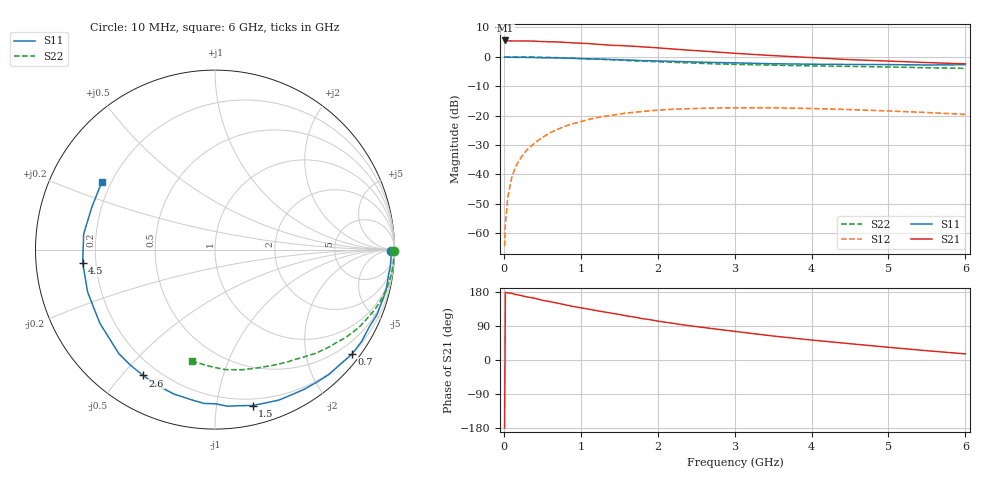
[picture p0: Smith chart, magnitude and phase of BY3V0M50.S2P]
! SIEMENS Small Signal Semiconductors
! BFY420
! Si NPN RF SIEGET Grounded Emitter Transistor in MICRO-X
! VCE = 3 V  IC = 0.5 mA
! Common Emitter S-Parameters:  October  1996
# GHz  S  MA  R  50
!  f  S11  S21  S12  S22
! GHz  MAG  ANG  MAG  ANG  MAG  ANG  MAG  ANG
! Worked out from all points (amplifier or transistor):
!   36 points, 10 MHz to 6 GHz, reference 50 ohm
!   highest |S21| = 5.6 dB at 20 MHz (marker M1)
!   |S21| within 3 dB of that: start of sweep to 2.243 GHz
!   unconditionally stable (mu >= 1): 4.71 GHz to end of sweep
!   at 250 MHz: K = 0.03, MSG = 19.3 dB, |S12| = -33.3 dB
!   at 1.4 GHz: K = 0.17, MSG = 11.9 dB, |S12| = -19.9 dB
!   at 6 GHz: K = 1.43, MAG = 4.7 dB, |S12| = -19.6 dB
!   S11 on the Smith chart (normalised r, x): 10 MHz: 81, -44; 700 MHz: 0.20, -2.96; 1.5 GHz: 0.15, -1.26; 2.6 GHz: 0.14, -0.57; 4.5 GHz: 0.15, -0.05; 6 GHz: 0.16, +0.27
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0.01  0.9811 -0.6  1.891 -179.2  0.0006 87.6  0.9999 -0.3
0.02  0.981 -1.2  1.897 178.8  0.0014 98.1  0.9999 -0.6
0.05  0.9817 -2.8  1.871 177.3  0.004 90.9  0.9999 -1.2
0.1  0.9812 -5.6  1.864 176.1  0.0086 88.0  0.9986 -2.5
0.15  0.9772 -8.1  1.861 172.7  0.0133 84.5  0.9964 -3.7
0.25  0.9793 -13.4  1.864 168.9  0.0217 81.1  0.9948 -6.2
0.4  0.9726 -21.7  1.847 163.0  0.0342 76.7  0.988 -9.9
0.5  0.9611 -26.9  1.813 157.6  0.0424 73.6  0.9821 -12.3
0.7  0.9604 -37.2  1.79 149.9  0.0585 66.8  0.9657 -17.1
0.9  0.9418 -47.6  1.727 141.3  0.0727 60.1  0.9451 -21.6
1.1  0.9231 -57.6  1.681 134.3  0.0858 54.2  0.9234 -25.9
1.5  0.8937 -76.4  1.558 120.2  0.1061 42.8  0.8786 -33.7
1.8  0.8592 -89.7  1.476 109.1  0.1172 35.2  0.8436 -39.0
2.2  0.8368 -105.8  1.356 96.7  0.1281 25.9  0.8072 -45.6
2.6  0.8074 -119.7  1.249 85.7  0.1331 18.1  0.7709 -51.5
3  0.7893 -132.7  1.147 75.6  0.1353 11.4  0.7448 -57.2
3.5  0.7614 -147.4  1.047 63.3  0.1357 4.4  0.7203 -63.6
4  0.7481 -161.4  0.969 52.7  0.1319 -1.5  0.7005 -70.2
4.5  0.7411 -174.3  0.894 43.0  0.1265 -6.3  0.6867 -77.1
5  0.7368 173.2  0.846 33.5  0.1198 -9.5  0.6716 -84.9
5.5  0.7258 161.1  0.798 24.5  0.1128 -11.7  0.6507 -92.7
6  0.7345 149.2  0.759 16.1  0.1046 -11.6  0.6351 -101.5
